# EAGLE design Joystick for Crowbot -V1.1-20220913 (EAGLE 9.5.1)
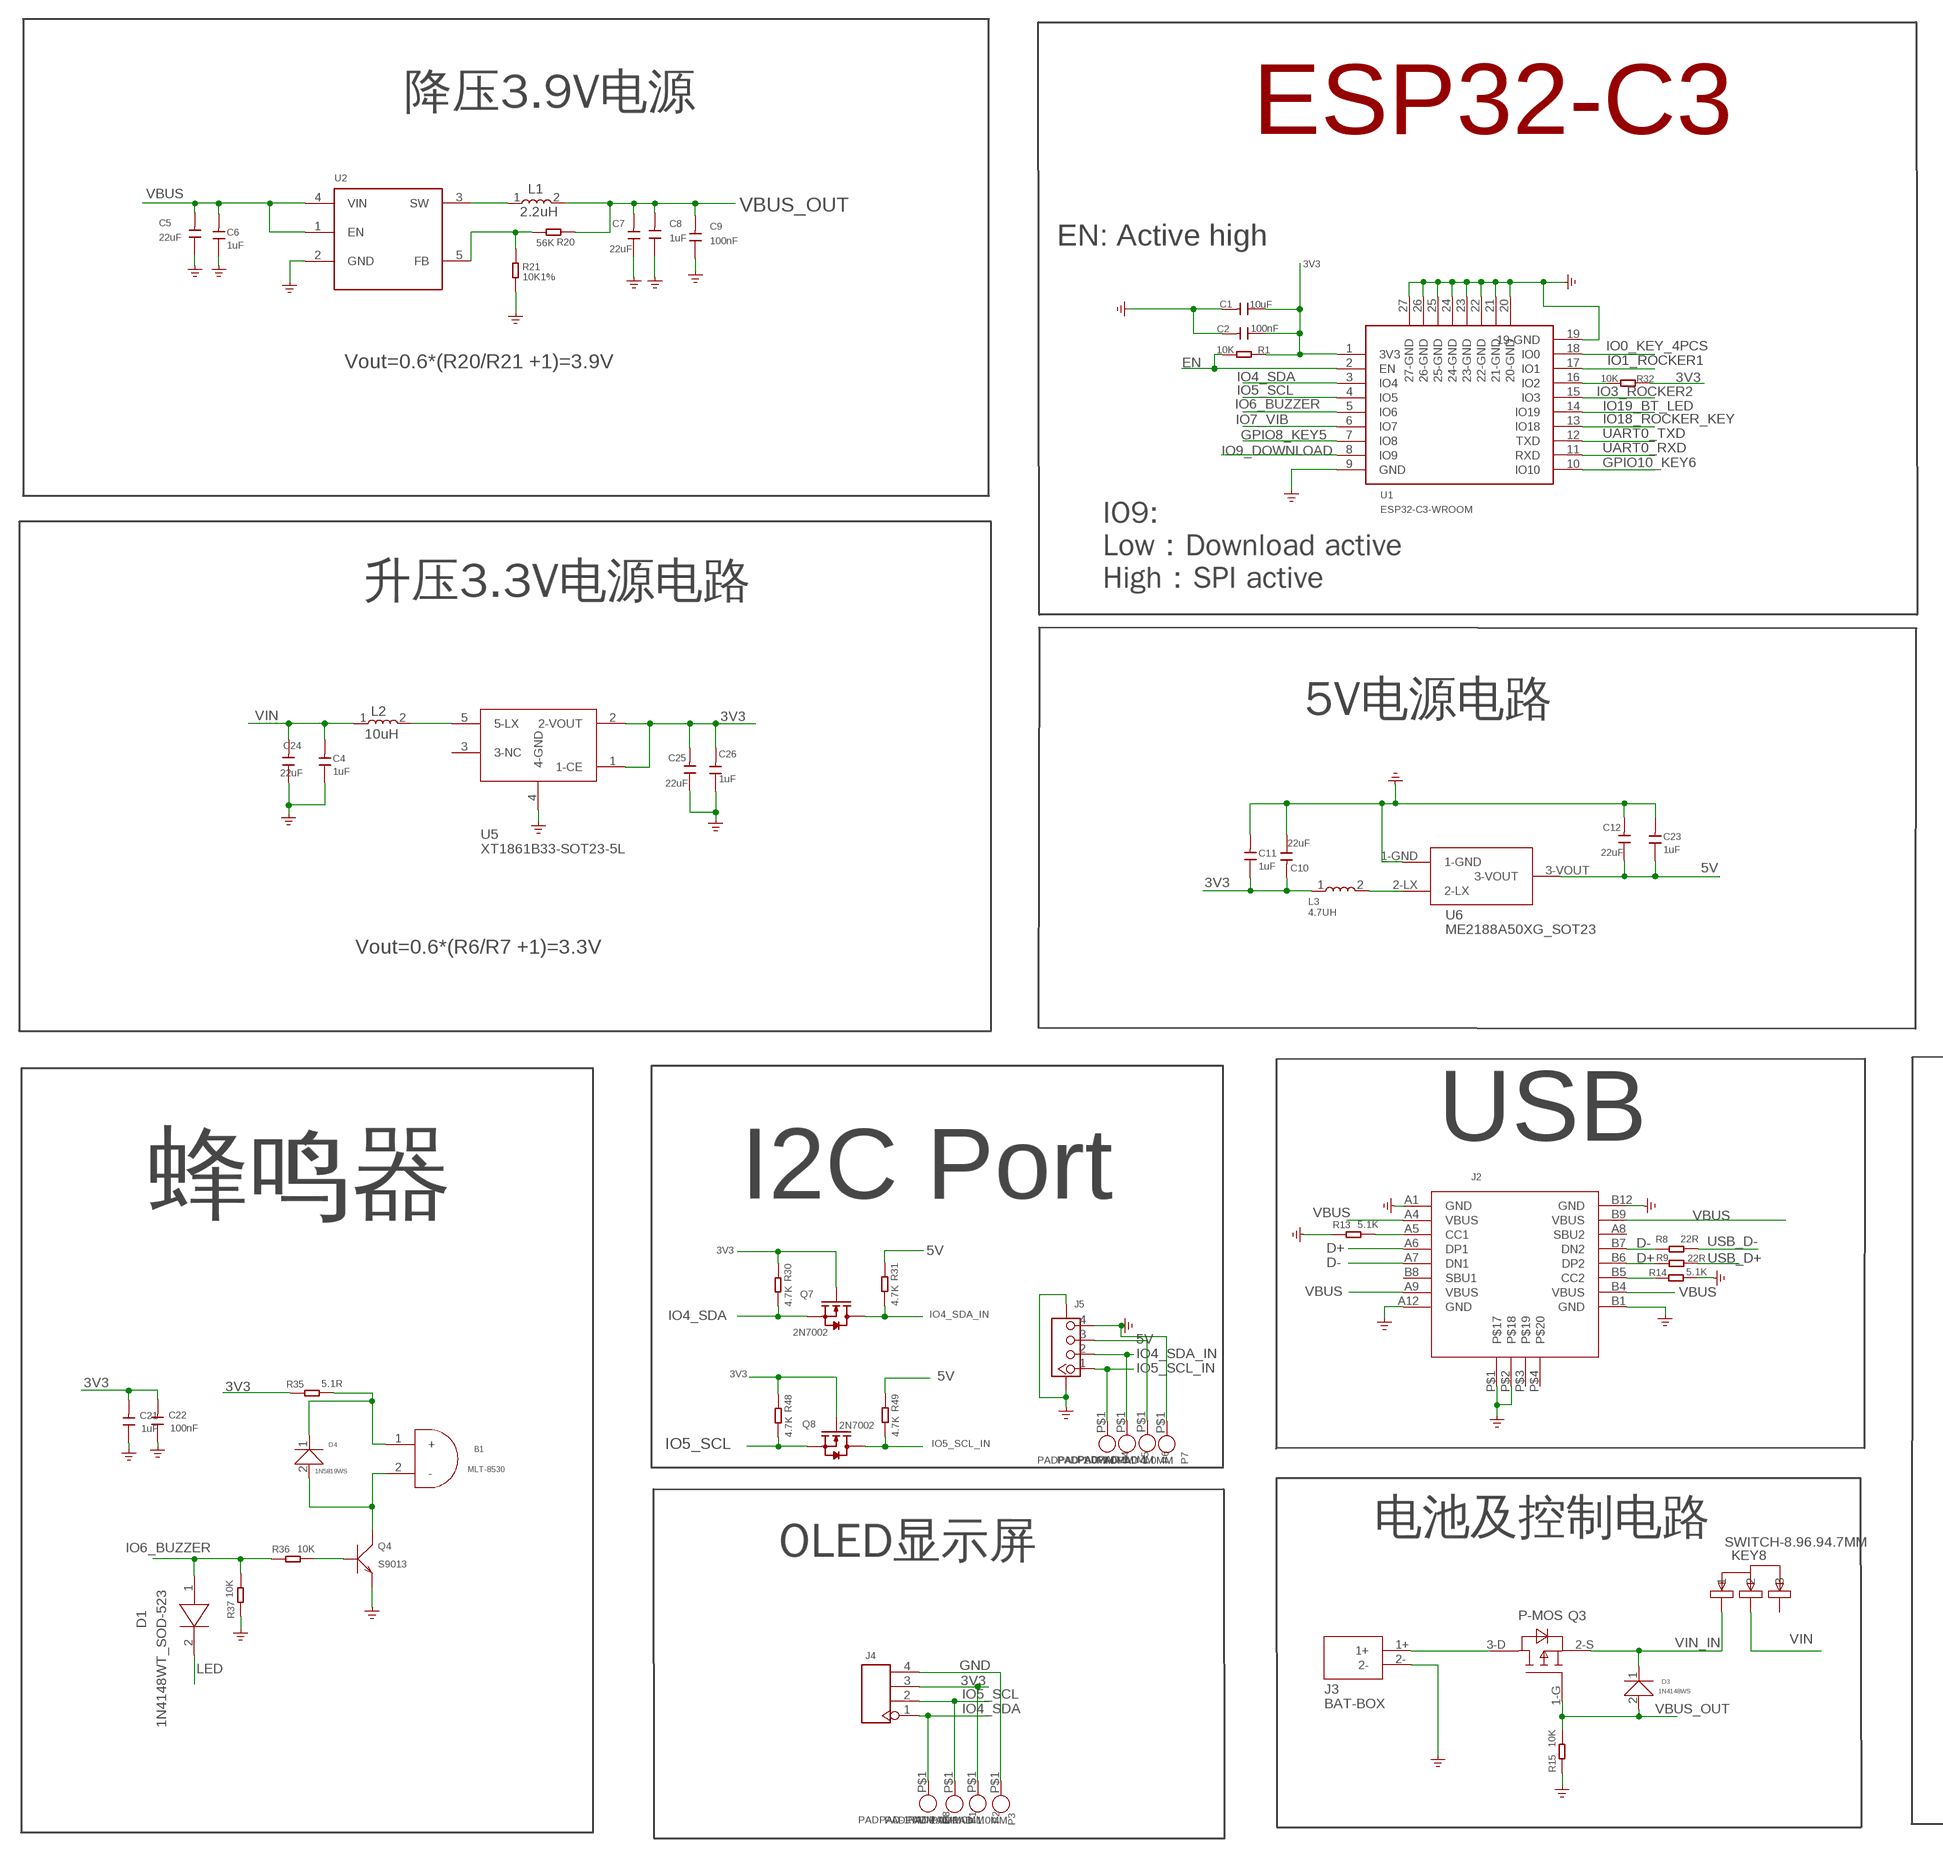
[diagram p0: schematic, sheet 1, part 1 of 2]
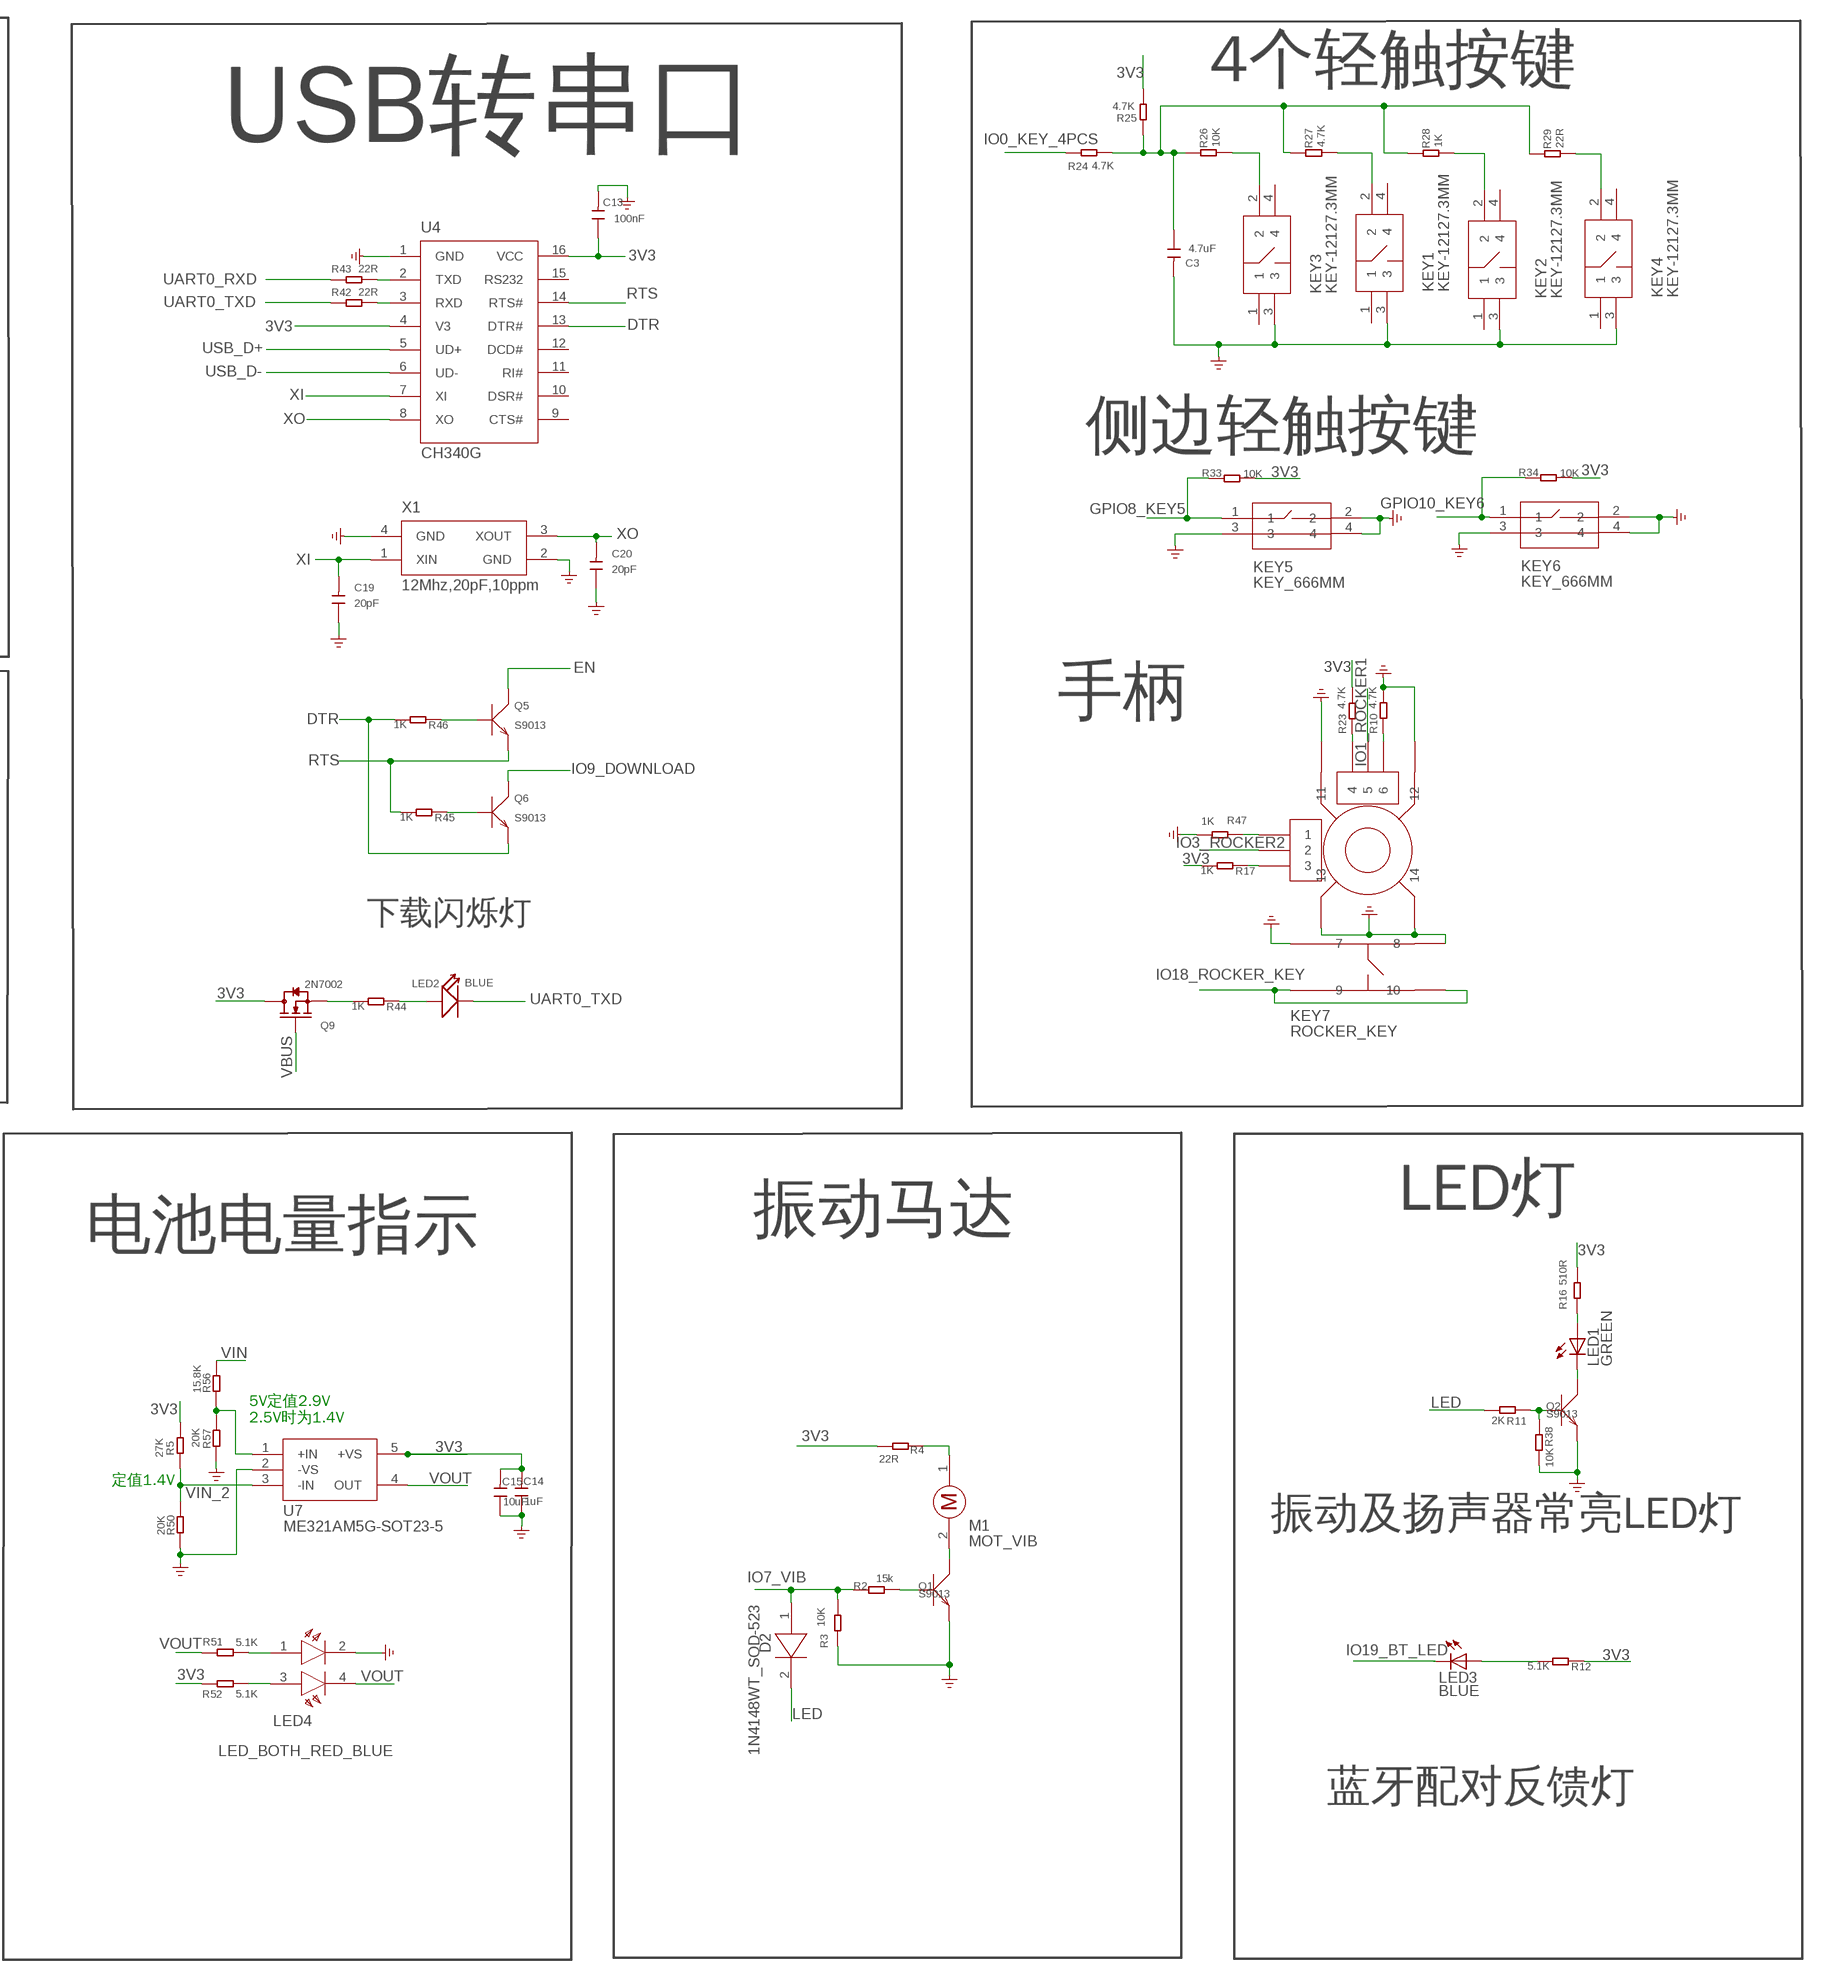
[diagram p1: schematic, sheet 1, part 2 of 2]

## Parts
B1  MLT-8530  [MLT-8530]
C1  10uF  DISCRETE_C-0603  [DISCRETE_C0603]
C2  100nF  DISCRETE_C-0603  [DISCRETE_C0603]
C3  4.7uF  C0603  [0603]
C4  1uF  C0603  [0603]
C5  22uF  C0805  [0805]
C6  1uF  C0603  [0603]
C7  22uF  C0805  [0805]
C8  1uF  C0603  [0603]
C9  100nF  C0603  [0603]
C10  22uF  C0805  [0805]
C11  1uF  C0603  [0603]
C12  22uF  C0805  [0805]
C13  100nF  C0603  [0603]
C14  1uF  DISCRETE_C-0603  [DISCRETE_C0603]
C15  10uF  DISCRETE_C-0603  [DISCRETE_C0603]
C19  20pF  C0603  [0603]
C20  20pF  C0603  [0603]
C21  1uF  DISCRETE_C-0603  [DISCRETE_C0603]
C22  100nF  DISCRETE_C-0603  [DISCRETE_C0603]
C23  1uF  C0603  [0603]
C24  22uF  C0805  [0805]
C25  22uF  C0805  [0805]
C26  1uF  C0603  [0603]
D1  1N4148WT_SOD-523  YSD200D5-30_SOD-523  [SOD-523]
D2  1N4148WT_SOD-523  YSD200D5-30_SOD-523  [SOD-523]
D3  1N4148WS  1N5819WS  [SOD-323]
D4  1N5819WS  [SOD-323]
J2  TYPEC-3.0-16P-SMD  [TYPEC-3.0-16P-SMD]
J3  BAT-BOX  [BAT-BOX]
J4  HEADER-4P-80/40MIL  [4P-2.54-80/40MIL]
J5  CONNECTOR_TWIG-4P-2.0-SMD-FEMALE-REINFORCE90D  [CONNECTOR_4P-SMD-2.0-90D]
KEY1  KEY-12127.3MM  [KEY-12*12*7.3MM]
KEY2  KEY-12127.3MM  [KEY-12*12*7.3MM]
KEY3  KEY-12127.3MM  [KEY-12*12*7.3MM]
KEY4  KEY-12127.3MM  [KEY-12*12*7.3MM]
KEY5  KEY_666MM  [KEY_6*6*6MM]
KEY6  KEY_666MM  [KEY_6*6*6MM]
KEY7  ROCKER_KEY  [ROCKER_KEY]
KEY8  SWITCH-8.96.94.7MM  [SWITCH-8.9*6.9*4.7MM]
L1  2.2uH  YP0403-L-SMD-4.5X4X3.2MM  [YP0403-L-SMD-4.5X4X3.2MM]
L2  10uH  YP0403-L-SMD-4.5X4X3.2MM  [YP0403-L-SMD-4.5X4X3.2MM]
L3  4.7UH  L_4.7UH  [L_2.5*2.0*1.2MM]
LED1  GREEN  LEDCHIP-LED0805  [CHIP-LED0805]
LED2  BLUE  DISCRETE_LED0603  [DISCRETE_LED-0603]
LED3  BLUE  LEDCHIP-LED0805  [CHIP-LED0805]
LED4  LED_BOTH_RED_BLUE  [LED_BOTH_RED_BLUE_SMD_1.6*1.6*0.6MM]
M1  MOT_VIB  [MOT_VIB]
P1  PADPAD-1.0MM  [PAD-1.0MM]
P2  PADPAD-1.0MM  [PAD-1.0MM]
P3  PADPAD-1.0MM  [PAD-1.0MM]
P4  PADPAD-1.0MM  [PAD-1.0MM]
P5  PADPAD-1.0MM  [PAD-1.0MM]
P6  PADPAD-1.0MM  [PAD-1.0MM]
P7  PADPAD-1.0MM  [PAD-1.0MM]
P8  PADPAD-1.0MM  [PAD-1.0MM]
Q1  S9013  TRANSISTOR-NPN-SOT23  [SOT23]
Q2  S9013  TRANSISTOR-NPN-SOT23  [SOT23]
Q3  P-MOS  CROWBOT-V1.0库_P-MOS  [CROWBOT-V1.0库_SOT-23]
Q4  S9013  TRANSISTOR-NPN-SOT23  [SOT23@1]
Q5  S9013  TRANSISTOR-NPN-SOT23  [SOT23@1]
Q6  S9013  TRANSISTOR-NPN-SOT23  [SOT23@1]
Q7  2N7002  MOSFET-N'SOT23'  [SOT23]
Q8  2N7002  MOSFET-N'SOT23'  [SOT23]
Q9  2N7002  MOSFET-N'SOT23'  [SOT23]
R1  10K  R0603  [R0603]
R2  15k  R-0603  [R0603]
R3  10K  R-0603  [R0603]
R4  22R  R-0603  [R0603]
R5  27K  R0603  [R0603]
R8  22R  DISCRETE_R-0603  [DISCRETE_R0603]
R9  22R  DISCRETE_R-0603  [DISCRETE_R0603]
R10  4.7K  DISCRETE_R-0603  [DISCRETE_R0603]
R11  2K  DISCRETE_R-0603  [DISCRETE_R0603]
R12  5.1K  DISCRETE_R-0603  [DISCRETE_R0603]
R13  5.1K  DISCRETE_R-0603  [DISCRETE_R0603]
R14  5.1K  DISCRETE_R-0603  [DISCRETE_R0603]
R15  10K  DISCRETE_R-0603  [DISCRETE_R0603]
R16  510R  DISCRETE_R-0603  [DISCRETE_R0603]
R17  1K  DISCRETE_R-0603  [DISCRETE_R0603]
R20  56K  DISCRETE_R-0603  [DISCRETE_R0603]
R21  10K1%  DISCRETE_R-0603  [DISCRETE_R0603]
R23  4.7K  DISCRETE_R-0603  [DISCRETE_R0603]
R24  4.7K  DISCRETE_R-0603  [DISCRETE_R0603]
R25  4.7K  DISCRETE_R-0603  [DISCRETE_R0603]
R26  10K  DISCRETE_R-0603  [DISCRETE_R0603]
R27  4.7K  DISCRETE_R-0603  [DISCRETE_R0603]
R28  1K  DISCRETE_R-0603  [DISCRETE_R0603]
R29  22R  DISCRETE_R-0603  [DISCRETE_R0603]
R30  4.7K  DISCRETE_R-0603  [DISCRETE_R0603]
R31  4.7K  DISCRETE_R-0603  [DISCRETE_R0603]
R32  10K  R0603  [R0603]
R33  10K  DISCRETE_R-0603  [DISCRETE_R0603]
R34  10K  DISCRETE_R-0603  [DISCRETE_R0603]
R35  5.1R  R0603  [R0603]
R36  10K  DISCRETE_R-0603  [DISCRETE_R0603]
R37  10K  DISCRETE_R-0603  [DISCRETE_R0603]
R38  10K  DISCRETE_R-0603  [DISCRETE_R0603]
R42  22R  DISCRETE_R-0603  [DISCRETE_R0603]
R43  22R  DISCRETE_R-0603  [DISCRETE_R0603]
R44  1K  DISCRETE_R-0603  [DISCRETE_R0603]
R45  1K  DISCRETE_R-0603  [DISCRETE_R0603]
R46  1K  DISCRETE_R-0603  [DISCRETE_R0603]
R47  1K  DISCRETE_R-0603  [DISCRETE_R0603]
R48  4.7K  DISCRETE_R-0603  [DISCRETE_R0603]
R49  4.7K  DISCRETE_R-0603  [DISCRETE_R0603]
R50  20K  R0603  [R0603]
R51  5.1K  DISCRETE_R-0603  [DISCRETE_R0603]
R52  5.1K  DISCRETE_R-0603  [DISCRETE_R0603]
R56  15.8K  R0603  [R0603]
R57  20K  R0603  [R0603]
U1  ESP32-C3-WROOM  [ESP32-C3-WROOM]
U2  A_XBJ_HM3420B  [A_XBJ_SOT23-5]
U4  CH340G  [SOP-16]
U5  XT1861B33-SOT23-5L  [XT1861B33-SOT23-5L]
U6  ME2188A50XG_SOT23  [ME2188A50XG_SOT23]
U7  ME321AM5G-SOT23-5  [ME321AM5G-SOT23-5]
X1  12Mhz,20pF,10ppm  XTAL  [SMD3225]

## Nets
3V3: C1.1 C2.1 C10.2 C11.1 C13.1 C14.2 C15.2 C21.2 C22.2 C25.2 C26.2 J4.3 L3.1 P2.P$1 Q7.1(G) Q8.1(G) Q9.3(D) R1.1 R4.2 R5.1 R12.1 R16.2 R17.2 R23.2 R25.2 R30.1 R32.1 R33.2 R34.2 R35.1 R48.1 R52.2 U1.1(3V3) U4.4(V3) U4.16(VCC) U5.1(1-CE) U5.2(2-VOUT) U7.5(+VS)
5V: C12.1 C23.1 J5.3 P6.P$1 R31.1 R49.1 U6.3-VOUT
D+: J2.A6(DP1) J2.B6(DP2) R9.1
D-: J2.A7(DN1) J2.B7(DN2) R8.1
DTR: Q6.2(E) R46.2 U4.13(DTR#)
EN: Q5.3(C) R1.2 U1.2(EN)
GND: C1.2 C2.2 C3.2 C4.1 C5.1 C6.1 C7.1 C8.1 C9.1 C10.1 C11.2 C12.2 C13.2 C14.1 C15.1 C19.1 C20.1 C21.1 C22.1 C23.2 C24.1 C25.1 C26.1 J2.A1(GND) J2.A12(GND) J2.B1(GND) J2.B12(GND) J2.P$1 J2.P$2 J3.2- J4.4 J5.4 J5.SS1 J5.SS2 KEY1.3 KEY2.3 KEY3.3 KEY4.3 KEY5.2 KEY5.3 KEY5.4 KEY6.2 KEY6.3 KEY6.4 KEY7.7 KEY7.8 KEY7.11 KEY7.12 KEY7.13 KEY7.14 LED4.2 P3.P$1 P7.P$1 Q1.2(E) Q2.2(E) Q4.2(E) R3.1 R10.2 R13.1 R14.2 R15.1 R21.2 R37.1 R38.2 R47.2 R50.2 R57.2 U1.9(GND) U1.19(19-GND) U1.20(20-GND) U1.21(21-GND) U1.22(22-GND) U1.23(23-GND) U1.24(24-GND) U1.25(25-GND) U1.26(26-GND) U1.27(27-GND) U2.2(GND) U4.1(GND) U5.4(4-GND) U6.1-GND U7.2(-VS) X1.2(GND) X1.4(GND)
GPIO8_KEY5: KEY5.1 R33.1 U1.7(IO8)
GPIO10_KEY6: KEY6.1 R34.1 U1.10(IO10)
IO0_KEY_4PCS: R24.1 U1.18(IO0)
IO1_ROCKER1: KEY7.5 U1.17(IO1)
IO3_ROCKER2: KEY7.2 U1.15(IO3)
IO4_SDA: J4.1 P8.P$1 Q7.2(S) R30.2 U1.3(IO4)
IO4_SDA_IN: J5.2 P5.P$1 Q7.3(D) R31.2
IO5_SCL: J4.2 P1.P$1 Q8.2(S) R48.2 U1.4(IO5)
IO5_SCL_IN: J5.1 P4.P$1 Q8.3(D) R49.2
IO6_BUZZER: D1.1 R36.1 R37.2 U1.5(IO6)
IO7_VIB: D2.1 R2.1 R3.2 U1.6(IO7)
IO9_DOWNLOAD: Q6.3(C) U1.8(IO9)
IO18_ROCKER_KEY: KEY7.9 KEY7.10 U1.13(IO18)
IO19_BT_LED: LED3.C U1.14(IO19)
LED: D1.2 D2.2 R11.2
N$1: L3.2 U6.2-LX
N$2: M1.2 Q1.3(C)
N$3: Q1.1(B) R2.2
N$4: M1.1 R4.1
N$5: L2.2 U5.5(5-LX)
N$6: B1.2(-) D4.2(+) Q4.3(C)
N$7: L1.1 U2.3(SW)
N$8: LED4.1 R51.2
N$9: LED1.A R16.1
N$10: KEY7.6 R10.1
N$11: J2.A5(CC1) R13.2
N$12: LED1.C Q2.3(C)
N$13: Q9.2(S) R44.2
N$14: B1.1(+) D4.1(-) R35.2
N$17: LED3.A R12.2
N$19: Q2.1(B) R11.1 R38.1
N$20: R20.2 R21.1 U2.5(FB)
N$21: J2.B5(CC2) R14.1
N$22: J3.1+ Q3.3-D(D)
N$23: C3.1 R24.2 R25.1 R26.1 R27.1 R28.1 R29.1
N$24: KEY4.2 R29.2
N$26: KEY2.2 R28.2
N$27: KEY3.2 R26.2
N$29: KEY1.2 R27.2
N$30: KEY7.1 R47.1
N$31: LED4.3 R52.1
N$32: Q5.1(B) R46.1
N$33: KEY7.4 R23.1
N$34: Q4.1(B) R36.2
N$35: KEY7.3 R17.1
N$36: R56.2 R57.1 U7.1(+IN)
N$38: Q6.1(B) R45.1
N$39: LED2.+ R44.1
N$40: R43.2 U4.2(TXD)
N$42: R42.2 U4.3(RXD)
N$53: R32.2 U1.16(IO2)
RTS: Q5.2(E) R45.2 U4.14(RTS#)
UART0_RXD: R43.1 U1.11(RXD)
UART0_TXD: LED2.- R42.1 U1.12(TXD)
USB_D+: R9.2 U4.5(UD+)
USB_D-: R8.2 U4.6(UD-)
VBUS: C5.2 C6.2 J2.A4(VBUS) J2.A9(VBUS) J2.B4(VBUS) J2.B9(VBUS) Q9.1(G) U2.1(EN) U2.4(VIN)
VBUS_OUT: C7.2 C8.2 C9.2 D3.2(+) L1.2 Q3.1-G(G) R15.2 R20.1
VIN: C4.2 C24.2 KEY8.2 L2.1 R56.1
VIN_2: R5.2 R50.1 U7.3(-IN)
VIN_IN: D3.1(-) KEY8.1 Q3.2-S(S)
VOUT: LED4.4 R51.1 U7.4(OUT)
XI: C19.2 U4.7(XI) X1.1(XIN)
XO: C20.2 U4.8(XO) X1.3(XOUT)
Unconnected: J2.A8(SBU2) J2.B8(SBU1) J2.P$3 J2.P$4 KEY1.1 KEY1.4 KEY2.1 KEY2.4 KEY3.1 KEY3.4 KEY4.1 KEY4.4 KEY8.3 U4.9(CTS#) U4.10(DSR#) U4.11(RI#) U4.12(DCD#) U4.15(RS232) U5.3(3-NC)

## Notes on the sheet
- 4个轻触按键
- 降压3.9V电源
- ESP32-C3 | USB转串口
- EN: Active high
- Vout=0.6*(R20/R21 +1)=3.9V
- 侧边轻触按键
- IO9:
  Low：Download active
  High：SPI active
- 升压3.3V电源电路
- 手柄
- 5V电源电路
- 下载闪烁灯
- Vout=0.6*(R6/R7 +1)=3.3V
- USB | LED灯
- 电池电量指示 | 振动马达
- 蜂鸣器 | I2C Port
- 5V定值2.9V
  2.5V时为1.4V
- 定值1.4V
- 振动及扬声器常亮LED灯
- 电池及控制电路
- OLED显示屏
- 蓝牙配对反馈灯

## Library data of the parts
B1 = A_xbj:MLT-8530
C1 C2 C14 C15 C21 C22 = A_xbj:DISCRETE_C*: Ceramic Capacitors
C3 C4 C6 C8 C9 C11 C13 C19 C20 C23 C26 = A_xbj:C0603
C5 C7 C10 C12 C24 C25 = A_xbj:C0805
D1 D2 = Joystick for Crowbot -V1.1-20220804:YSD200D5-30_SOD-523
D3 D4 = A_xbj:1N5819WS
J2 = A_xbj:TYPEC-3.0-16P-SMD
J3 = Crobot-Gamepad:BAT-BOX
J4 = Connector:HEADER-4P
J5 = A_xbj:CONNECTOR_TWIG-4P-2.0-SMD-FEMALE-REINFORCE
KEY1-KEY4 = Joystick for Crowbot -V1.1-20220804:KEY-12*12*7.3MM
KEY5 KEY6 = Joystick for Crowbot -V1.0-20220629:KEY_6*6*6MM
KEY7 = Joystick for Crowbot -V1.0-20220629:ROCKER_KEY
KEY8 = CrowBot -V1.2-20220707:SWITCH-8.9*6.9*4.7MM
L1 L2 = Joystick for Crowbot -V1.1-20220804:YP0403-L-SMD-4.5X4X3.2MM
L3 = CrowBOT-V1.0-20220530库:L_4.7UH
LED1 LED3 = led:LED: LED
LED2 = A_xbj:DISCRETE_LED*
LED4 = CrowBot_-V1.1-20220608:LED_BOTH_RED_BLUE
M1 = Joystick for Crowbot -V1.1-20220804:MOT_VIB
P1-P8 = crowpi_pow:PAD*
Q1 Q2 = Discrete:TRANSISTOR-NPN*: NPN audion
Q3 = CrowBot_-V1.1-20220617:CROWBOT-V1.0库_P-MOS
Q4-Q6 = discrete:TRANSISTOR-NPN*: NPN audion
Q7-Q9 = discrete:MOSFET-N: IRLL014: http://www.vishay.com/docs/91319/sihll014.pdf
R1 R32 R35 = A_xbj:R0603
R2-R4 = Discrete:R*
R5 R50 R56 R57 = cooper:R0603
R8-R17 R20 R21 R23-R31 R33 R34 R36-R38 R42-R49 R51 R52 = Crowtail-_LED-V2.0-20190615-01:DISCRETE_R*
U1 = Joystick for Crowbot -V1.1-20220804:ESP32-C3-WROOM
U2 = CrowBot_-V1.0-20220525:A_XBJ_HM3420B
U4 = A_xbj:CH340G
U5 = CrowBot_-V1.2-20220713:XT1861B33-SOT23-5L
U6 = Crobot-Gamepad:ME2188A50XG_SOT23
U7 = CrowBot_-V1.2-20220713:ME321AM5G-SOT23-5
X1 = A_xbj:XTAL

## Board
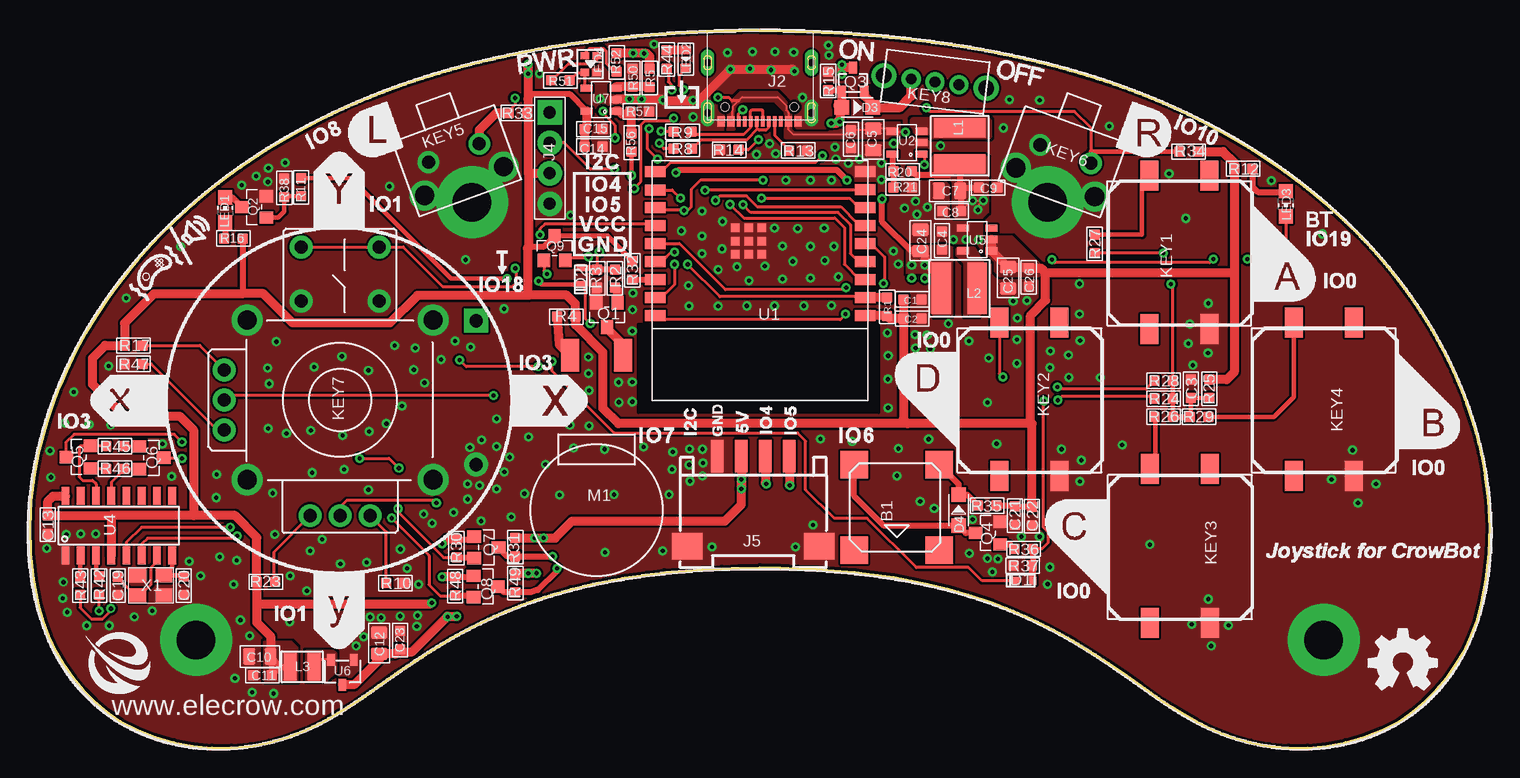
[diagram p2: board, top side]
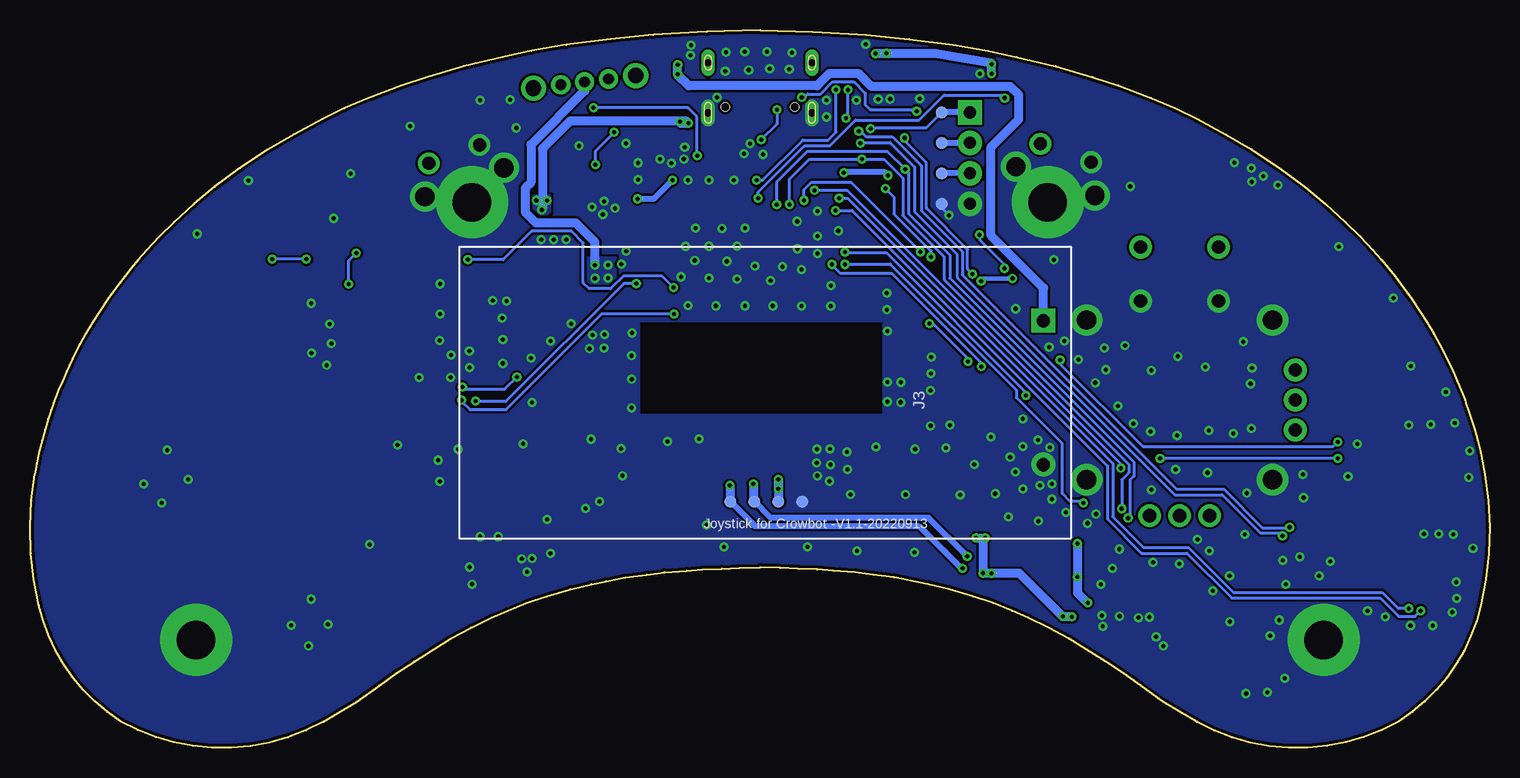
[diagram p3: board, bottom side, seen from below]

Size 121.68 x 59.85 mm. Coordinates in mm from the lower left corner, seen from the top.
Outline: 142 segments
Copper layers (1*16): Top 0.035mm / dielectric 1.5mm / Bottom 0.035mm
Design rules "default *": minimum track width 6mil, minimum drill 0.35mm, track to track 7mil, track to pad 7mil, pad to pad 7mil, via to via 7mil, smd to smd 7mil, copper to edge 10mil, drill to drill 6mil, minimum pad ring 10mil, minimum via ring 8mil, stop-mask expansion 4mil, vias tented up to drill 100mil, thermal gap 10mil
tRestrict: area 50.7,27.9 to 70.8,35.4
bRestrict: area 50.7,28 to 70.8,35.4

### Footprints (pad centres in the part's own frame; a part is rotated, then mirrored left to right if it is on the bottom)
MLT-8530 = smd 2.3 x 2.3: 1 -3.55,3.55; 2 -3.55,-3.55; 3 3.55,-3.55; 4 3.55,3.55
DISCRETE_C0603 = smd 0.889 x 0.889: 1 -0.762,0; 2 0.762,0
0603 = smd 0.889 x 0.889: 1 -0.762,0; 2 0.762,0
0805 = smd 1.016 x 1.397: 1 -0.889,0; 2 0.889,0
SOD-523 = smd 0.6 x 0.7: 1 -0.77,0; 2 0.65,0
SOD-323 = smd 1.2 x 1.2: 1 1.3,0; 2 -1.3,0
TYPEC-3.0-16P-SMD = smd 0.3 x 0.85: A1 -3.35,0; A4 -2.55,0; A5 -1.25,0; A6 -0.25,0; A7 0.25,0; A8 -1.75,0; A9 2.55,0; A12 3.35,0; B1 3.05,0; B4 2.25,0; B5 1.75,0; B6 0.75,0; B7 -0.75,0; B8 1.25,0; B9 -2.25,0; B12 -3.05,0 | drill 0.6 pad 1.016 long: P$1 -4.325,-0.72; P$2 4.325,-0.72; P$3 -4.325,-4.9; P$4 4.325,-4.9 | hole 0.68: -2.89,-1.22; 2.89,-1.22
BAT-BOX = drill 1.1 pad 2 square: 1+ -6.45,-0.2 | drill 1.1 pad 2: 2- 5.55,-0.2
4P-2.54-80/40MIL = drill 1.016 pad 2.032 square: 1 0,3.81 | drill 1.016 pad 2.032: 2 0,1.27; 3 0,-1.27; 4 0,-3.81
CONNECTOR_4P-SMD-2.0-90D = smd 1.01 x 2.74: 1 -3,-0.1; 2 -1,-0.1; 3 1,-0.1; 4 3,-0.1 | smd 2.54 x 2.184: SS1 -5.5,7.4; SS2 5.5,7.4
KEY-12*12*7.3MM = smd 2.5 x 1.5: 1 -5.8,2.5; 2 7,2.5; 3 -5.8,-2.5; 4 7,-2.5
KEY_6*6*6MM = drill 1.1 pad 1.8: 1 -2.35,-1.2; 2 2.15,-1.2 | drill 1.6 pad 2.5: 3 -3.6,1.3; 4 3.4,1.3
ROCKER_KEY = drill 1.1 pad 1.9: 1 2.5,-9.65; 2 0,-9.65; 3 -2.5,-9.65; 4 9.65,-2.5; 5 9.65,0; 6 9.65,2.5; 7 -8.25,-3.25; 8 -8.25,3.25; 9 -12.75,-3.25; 10 -12.75,3.25 | drill 1.6 pad 2.6: 11 6.65,-7.75; 12 6.65,7.75; 13 -6.65,-7.75; 14 -6.65,7.75
SWITCH-8.9*6.9*4.7MM = drill 0.9 pad 1.6: 1 -2.01,0; 2 -0.01,0; 3 1.99,0 | drill 1.3 pad 2.1: P$1 -4.31,0; P$2 4.29,0
YP0403-L-SMD-4.5X4X3.2MM = smd 4.3 x 1.6: 1 0,1.5; 2 0,-1.5
L_2.5*2.0*1.2MM = smd 1.1 x 2.3: 1 0,0; 2 2,0
CHIP-LED0805 = smd 1.2 x 1.2: A 0,-1.05; C 0,1.05
DISCRETE_LED-0603 = smd 0.762 x 0.889: + -0.762,0; - 0.762,0
LED_BOTH_RED_BLUE_SMD_1.6*1.6*0.6MM = smd 0.6 x 0.7: 1 -0.635,0.635; 2 0.765,0.635; 3 -0.635,-0.365; 4 0.765,-0.365
MOT_VIB = smd 1.5 x 2.7: 1 -2.2,12.9; 2 2.2,12.9
PAD-1.0MM = smd 1 x 1: P$1 0,0
SOT23 = smd 1.016 x 1.143: 1 -0.889,-1.016; 2 0.889,-1.016; 3 0,1.016
CROWBOT-V1.0库_SOT-23 = smd 0.7 x 1: 1-G -0.9,-0.8; 2-S 1,-0.8; 3-D 0.05,1.22
SOT23@1 = smd 1.016 x 1.143: 1 -0.95,-1.016; 2 0.95,-1.016; 3 0,1.016
R0603 = smd 0.889 x 0.889: 1 -0.762,0; 2 0.762,0
DISCRETE_R0603 = smd 0.889 x 0.889: 1 -0.762,0; 2 0.762,0
ESP32-C3-WROOM = smd 1.7 x 0.9: 1 -7.62,3.81; 2 -7.62,2.31; 3 -7.62,0.81; 4 -7.62,-0.69; 5 -7.62,-2.19; 6 -7.62,-3.69; 7 -7.62,-5.19; 8 -7.62,-6.69; 9 -7.62,-8.19; 10 9.88,-8.19; 11 9.88,-6.649; 12 9.88,-5.19; 13 9.88,-3.69; 14 9.88,-2.19; 15 9.88,-0.69; 16 9.88,0.81; 17 9.88,2.31; 18 9.88,3.81 | smd 0.7 x 0.7: 19 2.09,-2.39; 20 2.09,-3.49; 21 2.09,-1.29; 22 0.99,-1.29; 23 0.99,-2.39; 24 0.99,-3.49; 25 3.19,-1.29; 26 3.19,-2.39; 27 3.19,-3.49
A_XBJ_SOT23-5 = smd 0.6 x 1: 1 -0.95,-1.2; 2 0,-1.2; 3 0.95,-1.2; 4 0.95,1.2; 5 -0.95,1.2
SOP-16 = smd 0.66 x 1.5: 1 -4.445,-2.475; 2 -3.175,-2.475; 3 -1.905,-2.475; 4 -0.635,-2.475; 5 0.635,-2.475; 6 1.905,-2.475; 7 3.175,-2.475; 8 4.445,-2.475; 9 4.445,2.475; 10 3.175,2.475; 11 1.905,2.475; 12 0.635,2.475; 13 -0.635,2.475; 14 -1.905,2.475; 15 -3.175,2.475; 16 -4.445,2.475
XT1861B33-SOT23-5L = smd 0.6 x 1: 1 -0.95,-1.2; 2 0,-1.2; 3 0.95,-1.2; 4 0.95,1.2; 5 -0.95,1.2
ME2188A50XG_SOT23 = smd 0.635 x 1: 1-GND -0.95,-1; 2-LX 0.95,-1; 3-VOUT 0,1.1
ME321AM5G-SOT23-5 = smd 0.6 x 1: 1 -0.95,-1.2; 2 0,-1.2; 3 0.95,-1.2; 4 0.95,1.2; 5 -0.95,1.2
SMD3225 = smd 1.4 x 1.2: 1 -1.1,-0.85; 2 1.1,-0.85; 3 1.1,0.85; 4 -1.1,0.85

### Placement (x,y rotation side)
B1  72.25,20.04 270 top
C1  73.56,37.39 0 top
C2  73.56,35.8 0 top
C3  96.78,29.94 90 top
C4  76.01,42.29 270 top
C5  70.3,50.72 90 top
C6  68.44,50.75 90 top
C7  76.65,46.43 0 top
C8  76.82,44.73 0 top
C9  79.87,46.71 180 top
C10  19.16,7.61 0 top
C11  19.36,6.05 180 top
C12  29.1,8.72 90 top
C13  1.49,18.59 270 top
C14  46.98,50.14 180 top
C15  46.98,51.59 180 top
C19  7.32,13.5 90 top
C20  12.82,13.53 90 top
C21  82.1,19.36 90 top
C22  83.53,19.31 90 top
C23  30.85,8.99 90 top
C24  74.23,42.29 270 top
C25  81.53,39.19 90 top
C26  83.25,39.22 90 top
D1  82.83,13.92 180 top
D2  45.91,39.28 270 top
D3  68.95,53.39 0 top
D4  77.41,19.81 90 top
J2  60.82,52.22 180 top
J3  37,29.16 270 bottom
J4  43.32,49.18 0 top
J5  60.3,24.21 180 top
KEY1  KEY-1212*7.3MM  [KEY-12*12*7.3MM]  95.81,40.72 90 top
KEY2  KEY-1212*7.3MM  [KEY-12*12*7.3MM]  83.33,28.47 90 top
KEY3  KEY-1212*7.3MM  [KEY-12*12*7.3MM]  95.86,16.23 90 top
KEY4  KEY-1212*7.3MM  [KEY-12*12*7.3MM]  107.84,28.47 90 top
KEY5  KEY_66*6MM  [KEY_6*6*6MM]  35.65,48.44 200 top
KEY6  KEY_66*6MM  [KEY_6*6*6MM]  85.82,48.41 160 top
KEY7  25.85,29.01 270 top
KEY8  SWITCH-8.96.9*4.7MM  [SWITCH-8.9*6.9*4.7MM]  75.45,55.53 353 top
L1  77.51,50.19 0 top
L2  77.46,38.3 90 top
L3  21.68,6.76 0 top
LED1  16.27,44.86 0 top
LED2  54.68,57.43 270 top
LED3  104.69,45.37 180 top
LED4  46.6,57.07 270 top
M1  47.24,19.81 0 top
P1  45.7,50.45 0 bottom
P2  45.7,47.91 0 bottom
P3  45.7,45.37 0 bottom
P4  63.29,20.52 0 bottom
P5  61.29,20.52 0 bottom
P6  59.29,20.52 0 bottom
P7  57.29,20.52 0 bottom
P8  45.7,52.99 0 bottom
Q1  48.1,36.09 180 top
Q2  18.68,45.09 90 top
Q3  68.55,55.49 0 top
Q4  79.85,17.91 90 top
Q5  4.05,24.23 90 top
Q6  10.12,24.18 270 top
Q7  38.04,16.71 270 top
Q8  37.99,13.44 270 top
Q9  43.73,41.66 0 top
R1  71.45,36.77 90 top
R2  48.75,39.13 270 top
R3  47.28,39.13 90 top
R4  44.71,35.94 0 top
R5  51.66,55.84 270 top
R8  54.42,49.94 180 top
R9  54.4,51.36 180 top
R10  30.46,13.73 0 top
R11  22.6,46.74 90 top
R12  101.14,48.29 0 top
R13  64.02,49.81 180 top
R14  58.28,49.86 180 top
R15  66.54,55.6 270 top
R16  16.95,42.47 0 top
R17  8.64,33.54 180 top
R20  72.76,48.08 180 top
R21  72.76,46.71 0 top
R23  19.66,13.83 180 top
R24  94.5,29.11 0 top
R25  98.3,29.94 90 top
R26  94.5,27.6 180 top
R27  88.75,42.01 90 top
R28  94.5,30.61 180 top
R29  97.45,27.6 0 top
R30  35.55,16.63 270 top
R31  40.45,16.73 270 top
R32  50.21,39.82 270 top
R33  40.66,52.93 0 top
R34  96.59,49.71 0 top
R35  79.8,20.19 180 top
R36  82.83,16.59 180 top
R37  82.76,15.19 0 top
R38  21.2,46.69 90 top
R42  5.75,13.53 90 top
R43  4.18,13.53 90 top
R44  53.08,57.41 270 top
R45  7.1,25.15 180 top
R46  7.1,23.27 0 top
R47  8.64,32.02 180 top
R48  35.45,13.47 270 top
R49  40.45,13.72 270 top
R50  50.24,55.87 90 top
R51  44.21,55.65 180 top
R52  48.91,57.15 90 top
R56  50.15,50.46 90 top
R57  50.83,53.06 0 top
U1  61.99,39.85 180 top
U2  73.12,50.45 90 top
U4  7.41,18.52 0 top
U5  78.96,42.39 90 top
U6  26.06,6.35 180 top
U7  47.61,54.04 90 top
U$5  [SIG-2]  not placed on the board
U$9  [ELECROW-NEW]  4.6,4.48 0 top
U$56  [OSHW_FILLX200_NOTEXT]  111.6,4.83 0 top
X1  10.07,13.53 0 top

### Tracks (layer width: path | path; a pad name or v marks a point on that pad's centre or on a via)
3V3  (via drill 0.35)
  Top 0.406: R32.1 50.21,40.62 48.15,42.67 Q9.3 | 41.65,41.81 41.54,41.71 41.47,41.63
  Top 0.508: R35.1 82.02,20.19 C21.2 82.15,20.07 C22.2 | 1.7,20.77 1.93,20.99 | 6.7,19.36 6.77,19.28 | 41.57,37.73 41.54,37.76 41.47,37.83 | U7.5 45.02,54.48 41.87,54.48 41.54,54.15 | R48.1 36.87,14.23 Q8.1 | R30.1 36.82,17.39 Q7.1 | R23.2 18.9,12.02 | 33.42,12.02 v33.49,12.09 | 34.38,14.23 v34.36,14.25 | R16.2 17.71,37.88 17.72,37.87 | 41.54,41.81 42.87,41.81 Q9.3 | C11.1 20.84,6.76 L3.1 20.91,6.76 C10.2 20.13,7.54 C11.1
  Top 0.762: C14.2 C15.2 46.41,51.79 U7.5 | 41.54,47.88 43.3,47.88 J4.3 | R5.1 51.7,56.64 | U1.1 71.41,36.04 R1.1 71.66,35.8 C2.1 | C1.1 C2.1 | R34.2 99.46,49.71 100.38,48.78 R12.1 100.38,39.61 | 1.93,20.99 U4.16 | 1.7,20.77 1.49,20.55 C13.1 6.7,19.36 13.68,19.36 | 6.77,19.28 U4.4 | 13.68,19.36 17.08,19.36 18.9,17.54 R23.2 18.9,10.45 20.05,9.3 C10.2 | 41.57,37.73 44.74,37.73 45.47,37.01 R4.2 45.47,35.27 47.77,32.97 47.77,28.3 49.04,27.03 73.17,27.03 | 100.38,39.61 100.38,31.33 99.75,30.7 R25.2 | R52.2 51.37,57.91 51.66,57.62 R5.1 | 41.54,47.88 41.54,41.81 41.54,41.71 | 41.47,41.63 41.47,37.83 | 41.54,37.76 41.54,37.72 32.3,37.72 30,35.42 21.9,35.42 19.45,37.87 17.72,37.87 10.35,37.87 7.88,35.4 R17.2 6.26,33.54 5.2,32.48 5.2,30.33 7.86,27.66 12.46,27.66 13.63,26.49 13.63,19.41 13.68,19.36 | 41.54,47.88 41.54,52.88 | 41.54,52.88 41.54,54.15 41.51,54.12 41.51,56.21 v41.52,56.22 v41.52,57 v41.52,56.21 | 84.66,39.61 100.38,39.61 | C22.2 83.53,27.03 83.38,27.03 | 83.38,27.03 83.38,27.18 83.4,27.18 83.4,36.06 84.66,37.31 84.66,39.61 | R33.2 41.49,52.93 41.54,52.88 | R30.1 34.73,17.39 v34.36,17.02 | 18.9,12.02 33.42,12.02 | R48.1 34.38,14.23 | 83.38,27.03 73.17,27.03 | 73.17,27.03 72.8,27.4 C2.1 | U5.2 U5.1 C25.2 83.15,40.08 C26.2 84.29,39.98 84.66,39.61 | R5.1 51.66,57.65 51.42,57.89 v51.2,57.89
  Bottom 0.508: J4.3 P2.P$1 | 33.54,12.09 v33.49,12.09
  Bottom 0.762: v34.36,17.02 v34.36,14.25 34.36,12.9 33.54,12.09 | v50.28,57.91 51.17,57.91 v51.2,57.89 46.21,57.89 41.52,57.08 v41.52,56.21
  pour Top (no thermals): 79.72,42.67 81.85,42.67 84.22,40.31 84.22,39.4 84.11,39.29 80.86,39.29 80.43,39.73 80.43,40.51 79.95,41 79.72,41
  pour Top (no thermals): 19.52,8.87 21.78,8.87 22.21,8.43 22.29,8.36 22.29,5.56 22.24,5.51 19.7,5.51 19.52,5.69
5V  (via drill 0.35)
  Top 0.508: 59.32,22.43 59.3,22.4 | v59.3,22.38 | R49.1 40.53,14.56 | v42.23,14.56 v42.22,14.56
  Top 0.762: R31.1 v42.05,17.5 43.77,17.5 45.19,18.92 57.92,18.92 59.3,20.29 59.3,21.69 | 59.3,21.69 v59.3,22.38 59.3,22.4 | v42.22,14.56 40.53,14.56 | U6.3-VOUT 27.01,5.25 29.1,7.35 C12.1 30.46,7.83 C23.1 31.1,7.97 31.8,7.97 34.81,10.97 35.58,10.97 v35.58,10.95 | J5.3 59.32,24.28 59.32,22.43 | v59.3,22.38 59.3,21.7 59.3,21.69
  Bottom 0.762: P6.P$1 59.29,21.51 59.3,21.52 v59.3,22.38 v59.3,21.59 | v42.23,14.56 42.23,17.32 v42.05,17.5 42.81,17.5 v42.81,17.5 | v35.58,10.95 34.84,10.95 v34.81,10.92 35.58,10.92 39.21,14.56 v42.23,14.56 | v41.54,14.53 41.57,14.56 v42.23,14.56
D+
  Top 0.254: R9.1 55.18,51.36 55.41,51.14 59.49,51.14 60.08,51.72 J2.B6 60.07,53.1 60.16,53.19 61.03,53.19 61.07,53.14 J2.A6
D-
  Top 0.254: J2.B7 61.58,51.72 61.35,51.49 60.8,51.49 60.67,51.62 | 60.67,51.62 59.73,50.69 55.93,50.69 R8.1 | 60.67,51.62 60.57,51.72 J2.A7
DTR
  Top 0.254: Q6.2 7.9,23.23 R46.2 7.86,23.23 6.77,22.14 U4.13
EN  (via drill 0.35)
  Top 0.254: v12.66,25.5 12.03,26.14 3.67,26.14 3.04,25.5 Q5.3 | U1.2 69.15,37.54 69.08,37.62 57.52,37.62 v54.83,40.31 | v42.38,31.78 36.36,31.78 v35.8,32.34
  Top 0.762: R1.2 71.43,37.54 U1.2
  Bottom 0.254: v12.66,25.5 13.04,25.13 28.92,25.13 35.8,32.01 v35.8,32.34 | v54.83,40.31 54.83,40.26 54.15,39.58 49.88,39.58 42.38,32.07 v42.38,31.78
GND  (via drill 0.35, 3.2 pad 6)
  Top 0.762: Q1.2 47.21,38.29 R3.1 | U7.2 48.84,54.07 52.71,54.07 v52.77,54 52.85,53.93 55.21,53.93 v55.29,54 | v55.29,54 55.77,54 56.5,53.27 J2.P$2 | v55.29,54 55.79,54 v58.38,56.59 63.54,56.59 v63.72,56.41
  Bottom 0.254: P3.P$1 45.7,45.02 v45.07,44.4
  other vias: 107.84,8.99 84.84,45.49 36.84,45.49 13.84,8.99 42.48,56.21 55.29,52.6 64.4,54.23 61.66,50.37 68.21,48.74 67.1,50.09 67.17,49.1 70.98,47.37 62.17,49.53 66.82,47.32 65.06,47.32 63.01,47.32 73.83,45.57 74.82,45.09 73.93,44.48 72.91,44.98 60.01,56.62 61.76,56.52 58.16,57.96 60.24,58.04 62.09,58.04 63.67,57.99 21.27,48.79 19.83,47.19 19.88,48.34 18.86,47.68 17.64,46.91 56.07,24.89 56.1,23.75 56.05,22.68 54.98,24.92 54.96,23.6 55.03,22.23 65.27,18.59 63.82,16.74 56.86,16.74 52.75,16.41 75.38,19.97 84.17,17.6 82.64,17.6 74.21,20.55 72.28,22.68 72.41,24.94 80.58,25.35 74.92,25.73 68.54,25.55 110.71,20.42 112.21,22 110.25,24.82 108.5,22.38 99.91,10.21 98.47,8.48 96.84,10.29 98.24,12.4 98.24,37.06 81.96,37.24 83.1,37.29 82.31,35.84 82.26,34.04 82.26,32.06 79.92,32.49 78.27,33.91 76.57,35.36 85.05,33.07 85.03,31.7 86.58,32.74 86.6,30.89 87.54,33.96 89.25,30.86 96.94,31.9 96.56,33.71 98.21,32.92 96.69,35.33 53.58,24.66 53.53,23.22 2.78,13.82 2.73,12.45 3.11,11.3 8.7,10.92 6.59,10.19 4.74,10.19 10.18,11.41 14.21,14.33 13.27,15.55 1.39,16.64 3.04,17.78 4.23,17.83 5.48,17.83 4.92,26.95 6.75,26.9 6.57,31.83 42.97,23.62 66.82,36.88 65.9,25.76 62.07,36.86 64.51,36.86 69.15,49.07 70.98,48.77 75.91,50.19 72,50.39 72.38,40.34 79.06,42.37 18.3,9.32 17.54,10.64 16.98,13.62 17.08,5.79 18.53,4.62 20.31,4.52 32.25,10.14 30.85,10.97 32.32,11.02 29.28,10.85 27.8,9.25 28.36,10.9 27.19,8.48 62.07,43.33 64,43.31 62.73,41.83 67.02,41.81 66.21,43.33 81.14,51.69 66.61,57.76 66.56,58.57 60.57,49.48 74.79,34.42 73.78,34.47 75.05,33.28 73.83,33.33 80.69,15.75 79.82,15.77 78.3,16.21 80.23,14.66 78.58,19.05 39.54,22.99 38.9,25.12 37.66,25.66 36.49,22 38.9,21.59 37.48,21.87 39.97,24.23 19.85,26.62 23.41,26.47 28.26,26.37 19.8,31.67 23.69,31.75 28.21,31.47 31.99,31.52 23.36,16.41 20.41,17.78 15.81,15.93 21.66,10.52 31.43,14.96 32.4,13.62 30.88,16.56 87.65,23.98 85.99,24.89 87.52,22.2 85.03,15.06 84.83,13.64 39.51,36.6 35.45,33.91 36.72,33.43 34.28,32.39 32.12,33.33 33.52,18.72 35.32,19.64 36.49,20.73 52.01,58.68 84.17,54 89.98,51.84 94.96,47.88 103.47,47.3 107.74,42.85 12.56,41.78 8.02,37.49 3.65,29.67 26.18,23.22 23.51,22.94 20.23,21.24 15.56,22.78 15.51,20.85 11.8,22.63 1.74,22.56 1.67,24.77 71.97,41.43 87.49,38.69 87.49,36.17 96.36,44.15 93.36,16.94 79.82,28.78 50.21,30.51 41.57,25.91 29.96,46.81 36.31,40.69 91.05,25.25 32.88,30.43 31,28.5 29.71,27.03 38.9,27.43 36.67,25.05 32.81,19.48 28.06,15.47 25.87,15.34 21.68,14.33 23.08,13.08 2.91,27.08 11.04,25.32 47.51,54.13 26.05,26.04 21.38,26.21 19.93,30.35 20.54,33.86 26,32.64 30.39,33.53 28.21,21.51 24.35,17.37 17.24,15.62 37.61,18.9 40.12,19.25 47.94,16.28 81.65,54.05 49.98,54.1 50.97,54.08 65.06,41.81 63.59,40.56 61.25,40.16 62.73,39.09 65.06,39.17 66.26,40.64 67.4,39.27 59.93,38.96 57.37,39.88 56.02,41.2 57.7,41.61 57.72,43.89 56.02,44.76 56.02,42.67 54.29,43.1 58.94,40.11 54.93,36.83 54.9,38.53 59.76,36.86 50.26,37.92 50.23,36.53 50.21,34.75 50.21,28.86 49.06,30.48 49.09,28.8 46.57,31.22 51.15,25.07 47.89,24.89 45.33,24.99 45,26.9 46.55,32.59 53.28,21.11 48.68,21.11 44.13,21.08 41.21,21.18 46.6,29.8 46.6,26.85 71.49,34.6 71.54,32.69 71.52,30.74 71.54,28.35 57.37,36.83 78.02,42.37 76.98,42.37
  pour Bottom (rank 2, no thermals): -4.61,63.6 119.9,63.6 126.81,56.69 126.81,4.93 116.04,-5.84 -2.98,-5.84 -6.87,-1.95 -6.87,61.34
  pour Top (rank 2, no thermals): -4.05,63.15 124.17,63.15 130.88,56.44 130.88,-2.79 127.37,-6.3 -2.42,-6.3 -6.31,-2.41 -6.31,60.88
GPIO8_KEY5  (via drill 0.35)
  Top 0.254: U1.7 69.09,45.04 68.32,45.82 v60.98,45.82 | v40.43,54.18 40.43,53.62 39.89,53.09 R33.1
  Top 0.762: R33.1 38.87,52.93 37.45,51.51 KEY5.1
  Bottom 0.254: v60.98,45.82 60.98,46.33 57.1,50.2 55,50.2 52.87,52.34 47.57,52.34 45.48,54.43 40.68,54.43 v40.43,54.18
GPIO10_KEY6  (via drill 0.35)
  Top 0.254: v66.06,49.38 65.48,48.81 53.41,48.81 52.64,48.04 U1.10 | v74.72,53.37 75.02,53.06 87.08,53.06 88.44,51.71 KEY6.1
  Top 0.381: R34.1 88.44,49.71 KEY6.1
  Bottom 0.254: v66.06,49.38 66.08,49.38 66.08,52.61 66.84,53.37 v74.72,53.37
IO0_KEY_4PCS  (via drill 0.35)
  Top 0.254: U1.18 52.47,35.69 67.55,35.69 67.99,36.12 v67.99,36.17 | v85.69,28.98 85.99,29.29 93.56,29.29 R24.1
  Bottom 0.254: v67.99,36.17 68.01,36.2 73.98,36.2 81.98,28.2 85,28.2 85.69,28.88 v85.69,28.98
IO1_ROCKER1  (via drill 0.35)
  Top 0.254: v53.74,40.31 53.74,38.63 52.65,37.54 U1.17 | v33.87,20.42 33.68,20.61 26.38,20.61 25.85,20.08 KEY7.5
  Bottom 0.254: v53.74,40.31 53.71,40.34 49.98,40.34 39.46,29.82 39.46,29.19 35.68,25.41 35.68,21.24 35.02,20.58 34.03,20.58 v33.87,20.42
IO3_ROCKER2  (via drill 0.35)
  Top 0.254: U1.15 52.67,40.54 53.46,41.33 v53.74,41.33 | KEY7.2 16.55,29.36 v38.65,29.36
  Bottom 0.254: v53.74,41.33 53.69,41.28 50.29,41.28 38.65,29.64 v38.65,29.36
IO4_SDA  (via drill 0.35)
  Top 0.254: U1.3 69.15,39.04 67.88,40.31 67.88,43.38 67.1,44.17 59.5,44.17 v58.36,45.31 | v51.6,51.64 51.49,51.53 51.49,49.94 51.49,49.9 v52.31,49.07 | v30.67,19.94 30.67,19.66 34.46,15.87 R30.2
  Top 0.508: R30.2 36.97,15.87 Q7.2
  Bottom 0.254: v58.36,45.31 58.36,47.42 56.71,49.07 v52.31,49.07 50.49,49.07 48.92,47.51 48.92,44.38 45.49,40.95 45.49,39.04 30.09,23.64 30.09,22.93 30.67,22.35 v30.67,19.94 | P8.P$1 45.7,52.94 46.95,51.69 51.55,51.69 v51.6,51.64
  Bottom 0.508: J4.1 P8.P$1
IO4_SDA_IN  (via drill 0.35)
  Top 0.508: Q7.3 39.79,15.97 R31.2 43.53,15.97 v43.55,15.95
  Top 0.762: J5.2 61.3,22.08 v61.38,22
  Bottom 0.508: v43.55,15.95 46.78,19.18 59.94,19.18 P5.P$1
  Bottom 0.762: v61.38,22 61.38,20.62 P5.P$1
IO5_SCL  (via drill 0.35)
  Top 0.254: v59.43,45.29 60.07,44.64 67.36,44.64 68.39,43.61 68.39,41.23 69.07,40.54 U1.4 | v48.72,48.24 46.72,48.24 44.52,50.45 J4.2 | v30.14,19.15 33.26,16.03 33.26,13.59 34.2,12.65 35.39,12.65 R48.2
  Top 0.508: R48.2 36.82,12.71 Q8.2
  Bottom 0.254: v59.43,45.29 59.43,47.19 56.87,49.75 50.22,49.75 v48.72,48.24 48.44,47.97 48.44,44.54 45,41.1 45,39.16 29.65,23.81 29.65,22.66 29.99,22.33 29.99,19.3 v30.14,19.15
  Bottom 0.508: P1.P$1 J4.2
IO5_SCL_IN  (via drill 0.35)
  Top 0.508: 63.3,21.91 v63.34,21.87 | v43.93,14.96 43.93,14.76 42.33,13.15 41.75,12.96 R49.2 39.49,12.96 Q8.3
  Top 0.762: J5.1 63.3,21.91
  Bottom 0.508: 63.34,20.58 P4.P$1 61.25,18.49 47.58,18.49 43.99,14.9 v43.93,14.96
  Bottom 0.762: v63.34,21.87 63.34,20.58
IO6_BUZZER  (via drill 0.35)
  Top 0.254: U1.5 70.11,42.04 71.24,40.92 71.24,38.81 v71.14,38.71 | v84.52,28.91 84.44,28.83 84.44,18.42 84.85,18.01 84.85,17.07 84.37,16.59 R36.1
  Top 0.508: R36.1 83.6,16.58 D1.1 83.52,14.01 R37.2
  Bottom 0.254: v71.14,38.71 72.18,38.71 81.98,28.91 v84.52,28.91
IO7_VIB  (via drill 0.35)
  Top 0.254: v57.15,45.64 57.5,46 59.73,46 60.62,45.11 67.59,45.11 68.95,43.75 69.41,43.75 U1.6 | v47.46,41.35 47.43,41.35 47.28,41.2 R3.2
  Top 0.508: D2.1 47.12,40.05 R3.2 R2.1
  Bottom 0.254: v57.15,45.64 57.15,46.55 56.55,47.15 53.23,47.15 47.46,41.38 v47.46,41.35
IO9_DOWNLOAD  (via drill 0.35)
  Top 0.254: U1.8 69.56,46.49 v56.29,46.49 v56.28,46.48 | v30.75,23.32 29.92,24.14 29.91,24.13 v27.47,24.13 | Q6.3 12.61,24.18 v12.66,24.13
  Bottom 0.254: v56.28,46.48 v56.27,46.48 53.57,46.48 30.75,23.66 v30.75,23.32 | v12.66,24.13 v27.47,24.13
IO18_ROCKER_KEY  (via drill 0.35)
  Top 0.254: KEY7.9 KEY7.10 31.11,41.76 34.41,38.46 40.25,38.46 40.5,38.71 40.5,39.98 v40.45,39.98 | U1.13 51.98,43.67 42.92,43.67 42.53,43.28 v42.53,42.77
  Bottom 0.254: v42.53,42.77 42.53,42.37 40.45,40.29 v40.45,39.98
IO19_BT_LED  (via drill 0.35)
  Top 0.254: U1.14 54.14,42.04 57.98,38.2 67.86,38.2 v68.04,38.38 | v101.49,40.74 103.6,40.74 104.65,41.8 104.69,41.83 LED3.C | v85.18,40.7 85.43,40.45 98.35,40.45 v98.64,40.74
  Bottom 0.254: v68.04,38.38 69.03,39.37 72.17,39.37 73.27,38.28 75.07,38.28 75.55,38.76 75.55,42.09 76.55,43.08 79.85,43.08 82.23,40.7 v85.18,40.7 | v98.64,40.74 v101.49,40.74
LED  (via drill 0.35)
  Top 0.254: D1.2 79.36,13.92 78.25,15.04 73.88,15.04 69.79,19.13 67.05,19.13 64.66,21.51 64.66,25.58 63.99,26.25 48.7,26.25 43.5,31.45 v43.5,32.21 | D2.2 46.25,38.29 46.25,35.8 46.69,35.37 v46.71,35.37
  Top 0.381: R11.2 26.73,47.51 35.09,39.14 v39.77,39.14 | D2.2 42.66,38.63 v42.39,38.91
  Bottom 0.254: v46.71,35.37 46.41,35.37 43.49,32.45 43.49,32.22 v43.5,32.21
  Bottom 0.381: v42.39,38.91 42.16,39.14 v39.77,39.14
N$1
  Top 0.152: L3.2 24.3,7.38 25.08,7.38 U6.2-LX
  pour Top (no thermals): 23.08,8.13 25.29,8.13 25.52,7.9 25.52,6.35 24.7,5.54 23.13,5.54 23,5.67 23,8.05
N$2
  Top 0.762: Q1.3 48.1,34.97 49.44,33.63 M1.2
N$3
  Top 0.762: Q1.1 48.99,38.13 R2.2
N$4
  Top 0.762: M1.1 44.11,33.64 R4.1
N$5
  pour Top (no thermals): 77.41,41.73 78.68,41.73 79.67,40.04 79.67,36.6 79.03,35.97 77.99,35.97 77.89,36.07 77.89,40.39 77.23,41.05 77.23,41.56
N$6
  Top 0.508: Q4.3 78.01,17.91 D4.2 71.19,18.51 68.7,21 B1.2
N$7
  pour Top (no thermals): 73.62,52.53 79.9,52.53 80.1,52.33 80.1,50.9 80,50.8 75.22,50.8 75.15,50.88 75.15,51.11 75.12,51.13 73.85,51.13 73.45,51.54 73.45,52.35
N$8
  Top 0.254: R51.2 43.51,55.65 44.91,57.05 46.95,57.05 47.23,57.33 LED4.1
N$9
  Top 0.508: LED1.A 16.27,42.56 R16.1
N$10
  Top 0.254: R10.1 29.7,18.01 KEY7.6
N$11
  Top 0.254: J2.A5 62.07,51.08 63.26,49.89 R13.2
N$12
  Top 0.508: LED1.C 16.85,45.91 Q2.3
N$13  (via drill 0.35)
  Top 0.254: Q9.2 44.81,40.83 46.47,40.83 v46.57,40.94 | v50.38,46.64 50.38,46.66 50.93,47.22 50.93,51.94 51.29,52.3 53.46,52.3 v53.66,52.5 | R44.2 53.22,56.5 53.22,55.52 53.5,55.24 v53.5,54.86
  Bottom 0.254: v46.57,40.94 46.57,41.42 49.66,44.51 49.66,45.93 v50.38,46.64 | v53.5,54.86 53.53,54.83 53.53,52.63 v53.66,52.5
N$14
  Top 0.508: B1.1 77.41,21.99 D4.1 78.12,21.11 R35.2
N$17
  Top 0.508: R12.2 101.9,46.8 102.37,46.33 104.61,46.33 LED3.A
N$19
  Top 0.254: R38.1 21.26,45.98
  Top 0.381: Q2.1 20.7,44.2 21.2,44.71 R38.1 | 21.26,45.98 R11.1
N$20
  Top 0.508: U2.5 71.92,48.17 R20.2 R21.1
N$21  (via drill 0.35)
  Top 0.254: J2.B5 59.07,52.86 v59.42,53.2 | v60.72,50.7 59.88,49.86 R14.1
  Bottom 0.254: v59.42,53.2 59.42,52.01 v60.72,50.7
N$22  (via drill 0.35)
  Top 0.762: Q3.3-D 67.68,56.71 v67.68,56.16
  Bottom 0.762: J3.1+ 37.2,38.35 41.57,42.73 41.57,50.1 39.26,52.4 39.26,54.46 39.95,55.14 51.53,55.14 52.62,56.24 55.03,56.24 56.07,55.2 66.74,55.2 67.68,56.14 v67.68,56.16 v67.68,56.95
N$23  (via drill 0.35)
  Top 0.254: v94.48,41.25 R27.1 | v95.11,38.66 95.27,38.51 R28.1
  Top 0.381: R26.1 R24.2 R28.1 | R25.1 C3.1 96.78,27.69 R29.1
  Top 0.508: R26.1 R29.1
  Bottom 0.254: v95.11,38.66 95.11,40.62 v94.48,41.25
N$24
  Top 0.381: R29.2 103.69,27.6 105.34,29.25 KEY4.2
N$26  (via drill 0.35)
  Top 0.254: KEY2.2 80.8,35.45 80.8,31.2 v81.09,30.91 | v85.64,30.07 85.64,29.92 85.66,29.9 93.03,29.9 R28.2
  Bottom 0.254: v85.64,30.07 85.46,29.9 82.11,29.9 v81.09,30.91
N$27
  Top 0.381: R26.2 93.79,27.55 93.79,23.66 KEY3.2
N$29
  Top 0.381: KEY1.2 92.7,47.11 92.7,42.77 R27.2
N$30
  Top 0.254: R47.1 10.11,32.02 15.62,26.51 KEY7.1
N$31
  Top 0.254: LED4.3 46.23,57.92 46.63,58.31 47.81,58.31 48.03,58.09 48.03,57.06 48.71,56.39 R52.1
N$32
  Top 0.254: Q5.1 6.32,23.28 R46.1
N$33
  Top 0.254: R23.1 20.37,13.83 20.37,16.34 KEY7.4
N$34
  Top 0.508: Q4.1 81.7,16.96 R36.2
N$35
  Top 0.254: R17.1 14.16,33.54 KEY7.3
N$36
  Top 0.762: R56.2 50.12,51.26 50.12,53.01 R57.1 49.84,52.84 49.35,52.84 49.09,53.09 U7.1
N$38
  Top 0.254: Q6.1 7.88,25.13 R45.1
N$39
  Top 0.762: R44.1 53.1,58.19 LED2.+
N$40
  Top 0.381: R43.2 4.18,15.99 U4.2
N$42
  Top 0.381: R42.2 5.5,14.54 U4.3
N$53
  Top 0.508: R32.2 50.37,39.04 U1.16
RTS
  Top 0.254: R45.2 5.11,25.15 Q5.2 4.21,25.18 4.09,25.06 4.09,22.58 4.38,22.29 5.21,22.29 5.5,22 U4.14
UART0_RXD  (via drill 0.35)
  Top 0.254: U1.11 53.54,46.5 v54.22,45.82 | v6.75,11.61 6.75,11.43 6.06,10.75 5.12,10.75 4.18,11.69 R43.1
  Bottom 0.254: v6.75,11.61 7.61,11.61 8.95,12.95 21.35,12.95 25.1,16.7 28.86,16.7 31.42,19.27 31.42,23.71 53.53,45.82 v54.22,45.82
UART0_TXD  (via drill 0.35)
  Top 0.254: U1.12 52.31,44.84 54.52,44.84 v54.52,44.81 54.83,44.81 55.14,45.11 55.14,46.58 55.91,47.35 61.08,47.35 v61.1,47.32 | v5.76,11.43 R42.1 | v54.48,54.87 54.1,55.25 54.1,56.06 54.68,56.63 LED2.-
  Bottom 0.254: v5.76,11.43 6.24,10.95 7.58,10.95 9.12,12.48 21.5,12.48 25.24,16.22 29.02,16.22 31.86,19.07 31.86,23.52 53.15,44.81 v54.52,44.81 | v61.1,47.32 60.6,47.32 57.25,50.67 55.15,50.67 54.48,51.33 v54.48,54.87
USB_D+  (via drill 0.35)
  Top 0.254: R9.2 52.64,51.36 v52.59,51.41 | v16.68,18.39 9.3,18.39 8.04,17.13 U4.5
  Bottom 0.254: v52.59,51.41 52.44,51.41 51.98,50.95 49.8,50.95 47.39,48.54 47.39,44.8 43.96,41.38 43.96,39.43 26.11,21.58 22.17,21.58 18.93,18.34 16.73,18.34 v16.68,18.39
USB_D-  (via drill 0.35)
  Top 0.254: R8.2 52.85,49.94 52.47,50.32 v52.47,50.42 | U4.6 9.31,16.98 9.81,17.48 17.08,17.48 v17.26,17.65
  Bottom 0.254: v52.47,50.42 52.42,50.47 49.98,50.47 47.93,48.43 47.93,44.69 44.39,41.15 44.39,39.22 26.25,21.08 22.28,21.08 19.11,17.91 17.52,17.91 v17.26,17.65
VBUS  (via drill 0.35)
  Top 0.152: U2.4 71.85,51.46 71.7,51.61 C5.2 70.2,51.51 C6.2 68.06,51.13 63.64,51.13 63.24,51.54 63.24,52.09 | 63.24,52.09 J2.A4 J2.B9 | J2.A9 J2.B4 58.57,53.14 58.6,53.17 58.6,53.48 59.07,53.95 59.38,54.26 62.35,54.26 63.04,53.56 63.04,53.17 63.24,52.97 63.24,52.09
  Top 0.254: U2.1 74.55,49.27 v74.55,48.62 | v72.99,51.34 72.28,51.34 72.15,51.46 71.85,51.46 | Q9.1 42.84,39.78 v43.11,39.51 | 59.07,53.95 58.52,53.95 58.26,54.22 57.37,54.22 v57.35,54.23 | v47.76,53.09 47.76,52.91 48.77,51.9 v48.77,50.85
  Bottom 0.254: v72.99,51.34 72.99,51.29 74.55,49.73 v74.55,48.62 | v43.11,39.51 43.53,39.93 43.53,41.56 46.95,44.98 46.95,48.8 48.86,50.7 48.86,50.76 v48.77,50.85 | v57.35,54.23 57.13,54.23 56.86,54.51 55.78,54.51 54.77,55.53 53,55.53 52.06,54.58 52.06,53.62 51.62,53.19 47.85,53.19 v47.76,53.09
  pour Top (no thermals): 58.18,51.44 58.64,51.44 58.79,51.59 58.79,53.24 59.45,53.9 62.02,53.9 62.93,52.99 62.93,51.46 63.49,51.46 63.49,53.47 62.3,54.66 59.17,54.66 58.1,53.6 58.1,51.51
  pour Top (no thermals): 62.96,50.85 62.96,53.06 63.08,53.19 63.36,53.19 63.44,53.11 63.44,51.56 63.67,51.33 66.56,51.33 67.4,52.17 72.46,52.17 72.48,52.15 72.48,51.06 72.2,50.78 63.03,50.78
VBUS_OUT  (via drill 0.35)
  Top 0.152: 67.35,53.55 67.38,53.55 67.53,53.55 | 67.38,53.57 67.47,53.57 D3.2 | C8.2 78.48,45.62 v78.58,45.62 78.6,45.64 v79.47,45.64 79.01,45.19 v79.01,44.86
  Top 0.508: R20.1 73.86,47.75 76.57,47.75 L1.2 77.54,48.66 C7.2 77.59,46.38 | C9.2 77.59,46.71 77.59,46.38 | 77.59,46.38 C8.2 | R15.2 67.5,54.84 Q3.1-G
  Top 0.762: 67.38,53.57 67.38,53.55 | 67.53,53.55 67.53,52.4 67.2,52.07 v66.79,52.07 | Q3.1-G 67.65,53.85 67.35,53.55
  Bottom 0.762: v79.01,44.86 78.96,44.91 78.96,49.94 76.62,52.27 67,52.27 v66.79,52.07 67.43,52.07 67.5,52.15 v67.5,52.2
  pour Top (no thermals): 75.3,49.35 79.69,49.35 79.87,49.18 79.87,44.65 79.36,44.15 77.21,44.15 76.95,44.4 76.95,47.12 76.65,47.42 75.53,47.42 75.07,47.88 75.07,49.12
  pour Bottom (no thermals): 78.3,46.05 79.64,46.05 79.77,45.92 79.77,45.06 79.24,44.53 79.21,44.5 78.5,44.5 78.3,44.71
VIN  (via drill 0.35)
  Top 0.381: v50.15,47.73 R56.1
  Top 0.508: v71.03,45.77 71.03,43.84 73.47,41.4 C24.2 | v68.11,47.32 67.25,48.18 54.06,48.18 v53.84,47.96
  Top 0.762: C24.2 74.59,41.05 v74.59,40.26 74.9,40.26 75.96,39.19 L2.1
  Bottom 0.508: v71.03,45.77 69.66,45.77 v68.11,47.32 | v53.84,47.96 53.76,48.03 50.46,48.03 v50.15,47.73
  Bottom 0.762: KEY8.2 75.44,54.78 79.92,50.3 79.92,47.14 80.4,46.66 80.4,44.67 79.53,43.79 76.22,43.79 74.59,42.17 v74.59,40.26
  other vias: 74.59,39.14 73.5,40.26 73.5,39.17
  pour Top (no thermals): 73.09,41.89 76.85,41.89 76.85,36.09 76.67,35.92 75.48,35.92 75.15,36.25 75.15,39.29 74.87,39.57 73.09,39.57
  pour Bottom: 75.22,40.92 72.84,40.92 72.84,38.76 73.12,38.48 75.22,38.48
VIN_2
  Top 0.635: 48.81,55.07 U7.3
  Top 0.762: R5.2 51.64,55.11 R50.1 48.85,55.11 48.81,55.07
VIN_IN
  Top 0.762: Q3.2-S 69.55,54.36 70.25,53.66 D3.1 72.53,53.39 73.45,54.31 KEY8.1
VOUT
  Top 0.254: U7.4 46.23,55.17 LED4.4 45.63,56.31 R51.1
XI
  Top 0.254: C19.2 7.32,14.16 8.81,12.68 X1.1 9.05,12.6 10.09,13.64 10.09,15.03 10.58,15.52 U4.7
XO
  Top 0.381: C20.2 12.73,14.38 X1.3 11.85,15.06 U4.8

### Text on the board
tPlace: www.elecrow.com
bPlace: Joystick for Crowbot -V1.1-20220913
